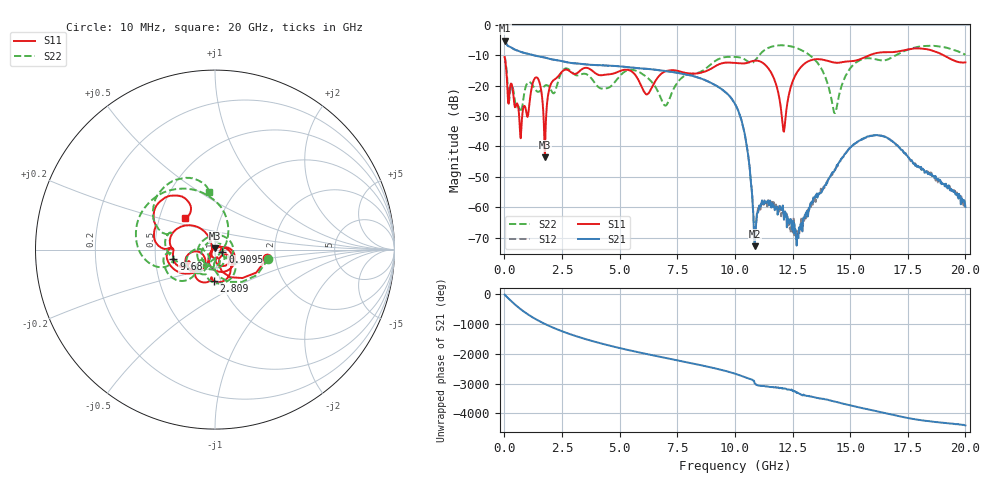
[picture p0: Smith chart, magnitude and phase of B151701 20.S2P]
!  2-Port S-parameters saved by WinCal
! VAR MeasName=S-Parameters (CALIBRATED_DATA) read from VNA (N5244A)
! VAR MeasDate=2015-12-24 19:10:29
! VAR NAME=B151701 20
! VAR FILENAME=B151701 20.S2P
! VAR DATE=2015-12-24 19:10:29
! VAR PHYS_PORTS=1,3
# Hz S DB R 50
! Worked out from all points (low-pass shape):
!   801 points, 10 MHz to 20 GHz, reference 50 ohm
!   highest |S21| = -5.20 dB at 10 MHz (marker M1); lowest = -72.8 dB at 10.85 GHz (marker M2)
!   |S21| within 3 dB of the highest: start of sweep to 454.1 MHz
!   lowest |S11| = -43.6 dB at 1.759 GHz (marker M3), VSWR 1.01, Z = 50 + j0.659 ohm
!   |S11| at or under -10 dB: start of sweep to 15.86 GHz; 19.04 GHz to end of sweep
!   |S22| runs from -29.1 to -6.8 dB; largest |S21 - S12| = 0.0014
!   S11 on the Smith chart (normalised r, x): 10 MHz: 1.81, -0.18; 909.5 MHz: 1.08, -0.03; 2.809 GHz: 0.93, -0.34; 9.68 GHz: 0.62, -0.07; 20 GHz: 0.68, +0.25
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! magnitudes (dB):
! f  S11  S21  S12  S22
! 10 MHz  -10.6  -5.2  -5.2  -10.4
! 584.7 MHz  -26.5  -8.6  -8.5  -26.8
! 909.5 MHz  -27.2  -9.4  -9.4  -20.8
! 1.409 GHz  -17.3  -10.3  -10.3  -21.9
! 1.759 GHz  -43.6  -10.8  -10.8  -20.0
! 2.034 GHz  -19.2  -11.3  -11.3  -21.6
! 2.809 GHz  -15.1  -12.5  -12.5  -14.8
! 3.358 GHz  -14.7  -12.9  -12.9  -16.2
! 6.182 GHz  -22.9  -14.5  -14.5  -17.3
! 6.682 GHz  -17.1  -14.9  -14.9  -22.3
! 9.68 GHz  -12.5  -22.8  -22.8  -10.6
! 10.01 GHz  -12.6  -26.0  -26.1  -10.6
! 10.48 GHz  -12.6  -38.2  -38.1  -11.7
! 10.85 GHz  -11.8  -72.8  -70.7  -11.9
! 11.63 GHz  -16.6  -58.7  -60.0  -7.1
! 12.13 GHz  -35.1  -64.1  -62.4  -6.8
! 12.7 GHz  -15.6  -69.7  -67.8  -7.8
! 13.35 GHz  -11.6  -58.5  -58.0  -10.7
! 14.33 GHz  -12.5  -47.7  -48.0  -29.1
! 15.15 GHz  -11.9  -39.3  -39.5  -13.1
! 16.68 GHz  -9.0  -37.6  -37.4  -11.3
! 20 GHz  -12.4  -59.9  -59.2  -9.9
